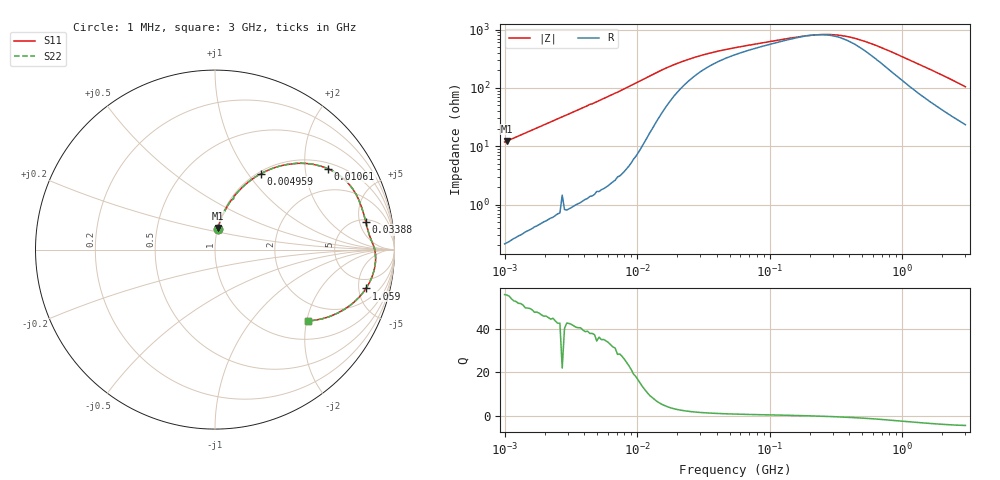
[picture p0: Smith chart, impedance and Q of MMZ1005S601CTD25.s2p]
! S-Parameter Data Generated by TDK Corporation
! Copyright(C) 2025 TDK Corporation.
! All Rights Reserved.
! TDK P/N: MMZ1005S601CTD25 (Chip Bead)
! Property: |Z|=600ohm at 100MHz
! Size(LxWxT): 1x0.5x0.5mm
! Model Type: s2p (Touchstone File Format Version 1.0)
! Frequency: DC=Yes Start=1MHz Stop=3000MHz 202points Log-sweep
! Model Generated on Feb. 6, 2025
! Terms and conditions regarding TDK Simulation Models:
! 1)This simulation model is being provided solely for informational
!  purposes. Please refer to the specifications of the products in
!  terms of detailed characteristics of such products.
! 2)In no event shall TDK Corporation of any of its subsidiaries be
!  liable for any loss or damage arising, directly or indirectly,
!  from any information contained in this simulation model, including,
!  but not limited to loss or damages arising from any inaccuracies,
!  omissions or errors in connection with such information.
! 3)Any and all copyrights on this simulation model are owned by
!  TDK Corporation.  Duplication or redistribution of this simulation
!  model without prior written permission from TDK Corporation
!  is prohibited.
! 4)This simulation model is subject to any modification or change
!  without any prior notice.
! 5)Neither TDK Corporation nor any of its subsidiaries shall make any
!  warranty, express or implied, including but not limited to the
!  correctness, implied warranties of merchantability and fitness for
!  a particular purpose with respect to this simulation models.
! 6)The use of this simulation model shall be deemed to have consented
!  to the terms and conditions hereof.
! Port Assignments:
!  1 ---@@@--- 2
! Applicable Conditions:
!  Temperature = 25 degC
!  DC Bias Current = 0 A
!  Small Signal Operation
# Hz S MA R 50
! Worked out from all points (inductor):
!   201 points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, 1 MHz to 3 GHz, reference 50 ohm
!   read as one part in series: L = 1.87 uH near 1.041 MHz
!   highest Q = 55.5 at 1.041 MHz (marker M1), where L = 1.87 uH
!   self-resonance near 217.2 MHz
!   S11 on the Smith chart (normalised r, x): 1 MHz: 1.00, +0.24; 4.959 MHz: 1.03, +1.16; 10.61 MHz: 1.18, +2.65; 33.88 MHz: 5.50, +6.24; 1.059 GHz: 3.41, -6.02; 3 GHz: 1.47, -2.03
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1000000  0.1167 82.3  0.9911 -6.7  0.9911 -6.7  0.1167 82.3
1040844  0.1214 82.0  0.9904 -7.0  0.9904 -7.0  0.1214 82.0
2226959  0.2509 74.2  0.9624 -14.5  0.9624 -14.5  0.2509 74.2
2947212  0.323 69.8  0.9389 -18.8  0.9389 -18.8  0.323 69.8
3900413  0.4119 64.2  0.9008 -24.3  0.9008 -24.3  0.4119 64.2
4959344  0.4944 58.7  0.855 -29.6  0.855 -29.6  0.4944 58.7
7400828  0.6507 47.4  0.7368 -40.6  0.7368 -40.6  0.6507 47.4
8686058  0.711 42.2  0.673 -45.3  0.673 -45.3  0.711 42.2
1.061086e7  0.7747 35.5  0.5823 -50.6  0.5823 -50.6  0.7747 35.5
1.461624e7  0.8335 25.3  0.4338 -55.3  0.4338 -55.3  0.8335 25.3
2.013356e7  0.8488 17.8  0.3224 -53.5  0.3224 -53.5  0.8488 17.8
3.387922e7  0.8538 10.4  0.222 -43.8  0.222 -43.8  0.8538 10.4
5.477226e7  0.86 6.6  0.1761 -34.1  0.1761 -34.1  0.86 6.6
2.136344e8  0.8896 0.1  0.1105 -0.7  0.1105 -0.7  0.8896 0.1
2.827291e8  0.894 -1.5  0.1087 12.0  0.1087 12.0  0.894 -1.5
3.741707e8  0.8966 -3.3  0.1166 25.9  0.1166 25.9  0.8966 -3.3
5.364635e8  0.8956 -6.2  0.1458 41.3  0.1458 41.3  0.8956 -6.2
8.005644e8  0.8859 -10.5  0.2061 51.3  0.2061 51.3  0.8859 -10.5
1.059487e9  0.8689 -14.4  0.268 53.8  0.268 53.8  0.8689 -14.4
1.782824e9  0.7993 -24.2  0.4248 50.4  0.4248 50.4  0.7993 -24.2
2.266846e9  0.7433 -29.9  0.5136 46.2  0.5136 46.2  0.7433 -29.9
3e9  0.6525 -37.6  0.6256 39.5  0.6256 39.5  0.6525 -37.6
